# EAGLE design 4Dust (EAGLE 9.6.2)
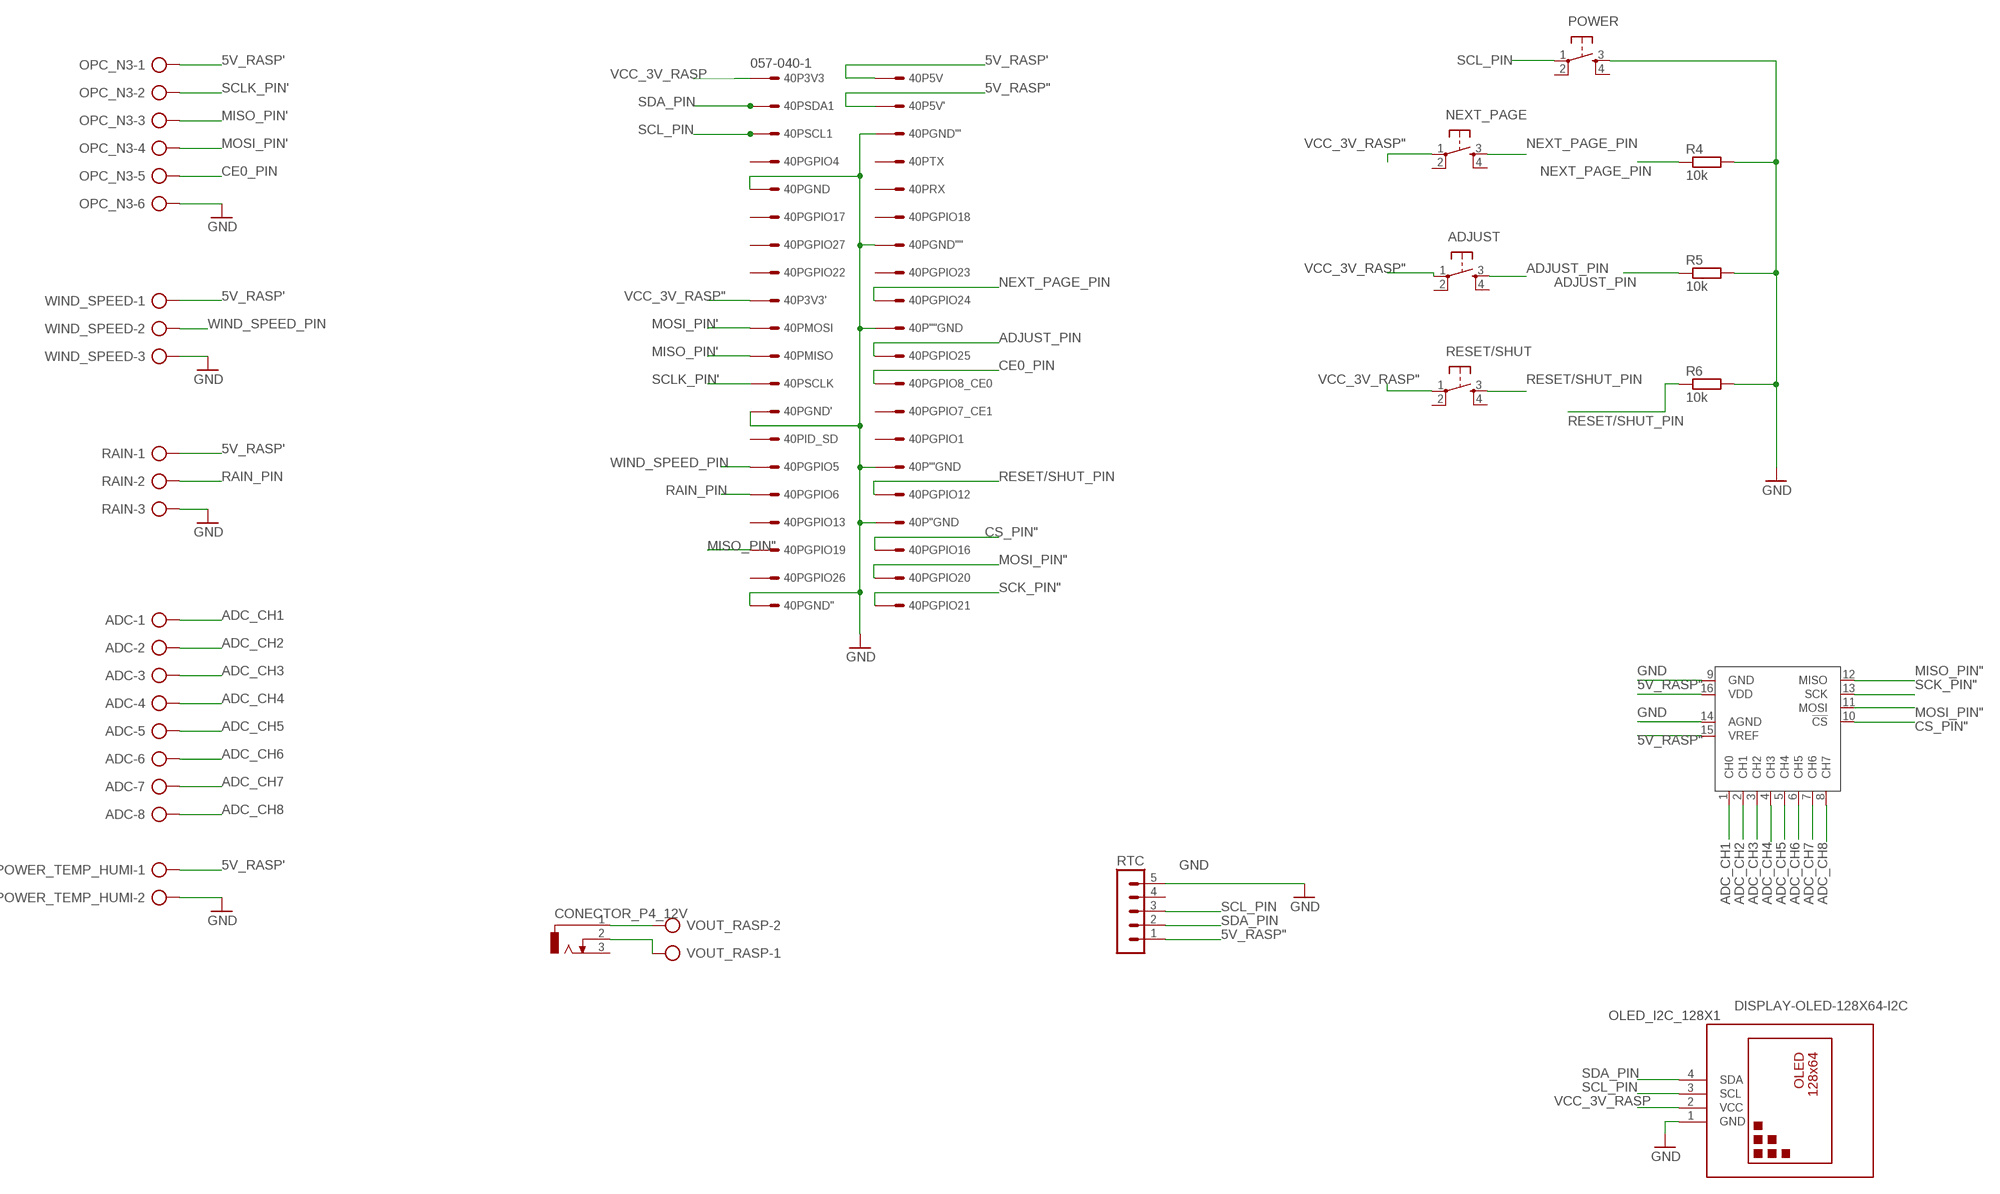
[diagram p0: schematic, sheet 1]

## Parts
40P  057-040-1  [057-040-1]
ADC  AK500/8  [AK500/8]
ADJUST  TAC_SWITCHPTH  [TACTILE-PTH]
CONECTOR_P4_12V  DCJ0303  [DCJ0303]
MCP3008  MCP3008P  [DIL16]
NEXT_PAGE  TAC_SWITCHPTH  [TACTILE-PTH]
OLED_I2C_128X1  DISPLAY-OLED-128X64-I2C  [DISPLAY-OLED-128X64-I2C]
OPC_N3  AK500/6  [AK500/6]
POWER  TAC_SWITCHPTH  [TACTILE-PTH]
POWER_TEMP_HUMI  AK500/2  [AK500/2]
R4  10k  R-EU_0204/7  [0204/7]
R5  10k  R-EU_0204/7  [0204/7]
R6  10k  R-EU_0204/7  [0204/7]
RAIN  AK500/3  [AK500/3]
RESET/SHUT  TAC_SWITCHPTH  [TACTILE-PTH]
RTC  MA05-1  [MA05-1]
VOUT_RASP  AK500/2  [AK500/2]
WIND_SPEED  AK500/3  [AK500/3]

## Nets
5V_RASP": 40P.4 MCP3008.15(VREF) MCP3008.16(VDD) RTC.1
5V_RASP': 40P.2 OPC_N3.1 POWER_TEMP_HUMI.1 RAIN.1 WIND_SPEED.1
ADC_CH1: ADC.1 MCP3008.1(CH0)
ADC_CH2: ADC.2 MCP3008.2(CH1)
ADC_CH3: ADC.3 MCP3008.3(CH2)
ADC_CH4: ADC.4 MCP3008.4(CH3)
ADC_CH5: ADC.5 MCP3008.5(CH4)
ADC_CH6: ADC.6 MCP3008.6(CH5)
ADC_CH7: ADC.7 MCP3008.7(CH6)
ADC_CH8: ADC.8 MCP3008.8(CH7)
ADJUST_PIN: 40P.22 ADJUST.3 R5.1
CE0_PIN: 40P.24 OPC_N3.5
CS_PIN": 40P.36 MCP3008.10(!CS)
GND: 40P.6 40P.9 40P.14 40P.20 40P.25 40P.30 40P.34 40P.39 MCP3008.9(GND) MCP3008.14(AGND) OLED_I2C_128X1.1(GND) OPC_N3.6 POWER.3 POWER_TEMP_HUMI.2 R4.2 R5.2 R6.2 RAIN.3 RTC.5 WIND_SPEED.3
MISO_PIN": 40P.35 MCP3008.12(MISO)
MISO_PIN': 40P.21 OPC_N3.3
MOSI_PIN": 40P.38 MCP3008.11(MOSI)
MOSI_PIN': 40P.19 OPC_N3.4
N$1: CONECTOR_P4_12V.1 VOUT_RASP.2
N$2: CONECTOR_P4_12V.2 VOUT_RASP.1
NEXT_PAGE_PIN: 40P.18 NEXT_PAGE.3 R4.1
RAIN_PIN: 40P.31 RAIN.2
RESET/SHUT_PIN: 40P.32 R6.1 RESET/SHUT.3
SCK_PIN": 40P.40 MCP3008.13(SCK)
SCL_PIN: 40P.5 OLED_I2C_128X1.3(SCL) POWER.1 RTC.3
SCLK_PIN': 40P.23 OPC_N3.2
SDA_PIN: 40P.3 OLED_I2C_128X1.4(SDA) RTC.2
VCC_3V_RASP: 40P.1 OLED_I2C_128X1.2(VCC)
VCC_3V_RASP": 40P.17 ADJUST.1 NEXT_PAGE.1 RESET/SHUT.1
WIND_SPEED_PIN: 40P.29 WIND_SPEED.2
Unconnected: 40P.7 40P.8 40P.10 40P.11 40P.12 40P.13 40P.15 40P.16 40P.26 40P.27 40P.28 40P.33 40P.37 ADJUST.2 ADJUST.4 CONECTOR_P4_12V.3 NEXT_PAGE.2 NEXT_PAGE.4 POWER.2 POWER.4 RESET/SHUT.2 RESET/SHUT.4 RTC.4

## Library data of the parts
40P = con-panduit-40pin_header:057-040-: CONNECTOR 40-pin series 057 contact pc board low profile headers; OC_FARNELL: unknown; OC_NEWARK: unknown
ADC = con-ptr500:AK500/8: CONNECTOR; OC_FARNELL: unknown; OC_NEWARK: unknown
ADJUST NEXT_PAGE POWER RESET/SHUT = SparkFun:TAC_SWITCH: Momentary Switch Button commonly used for reset or general input. Spark Fun Electronics SKU : COM-00097
CONECTOR_P4_12V = con-jack:DCJ0303: DC POWER JACK Source: DCJ0303.pdf; OC_FARNELL: unknown; OC_NEWARK: unknown
MCP3008 = MCP3008:MCP3008
OLED_I2C_128X1 = diy-modules:DISPLAY-OLED-128X64-I2C: 128x64 Dot Matrix OLED Module based on SSD1306 chip Variant with I2C interface More details available here: http://www.instructables.com/id/Monochrome-096-i2c-OLED-display-with-arduino-SSD13/ SSD1306 datasheet: https://cdn-shop.adafruit.com/datasheets/SSD1306.pdf Click here to find device on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
OPC_N3 = con-ptr500:AK500/6: CONNECTOR; OC_FARNELL: unknown; OC_NEWARK: unknown
POWER_TEMP_HUMI VOUT_RASP = con-ptr500:AK500/2: CONNECTOR; OC_FARNELL: unknown; OC_NEWARK: unknown
R4-R6 = rcl:R-EU_: RESISTOR, European symbol; SPICEPREFIX: R
RAIN WIND_SPEED = con-ptr500:AK500/3: CONNECTOR; OC_FARNELL: unknown; OC_NEWARK: unknown
RTC = con-lstb:MA05-1: PIN HEADER; OC_FARNELL: unknown; OC_NEWARK: unknown

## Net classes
0 default: clearance 0.205 mm

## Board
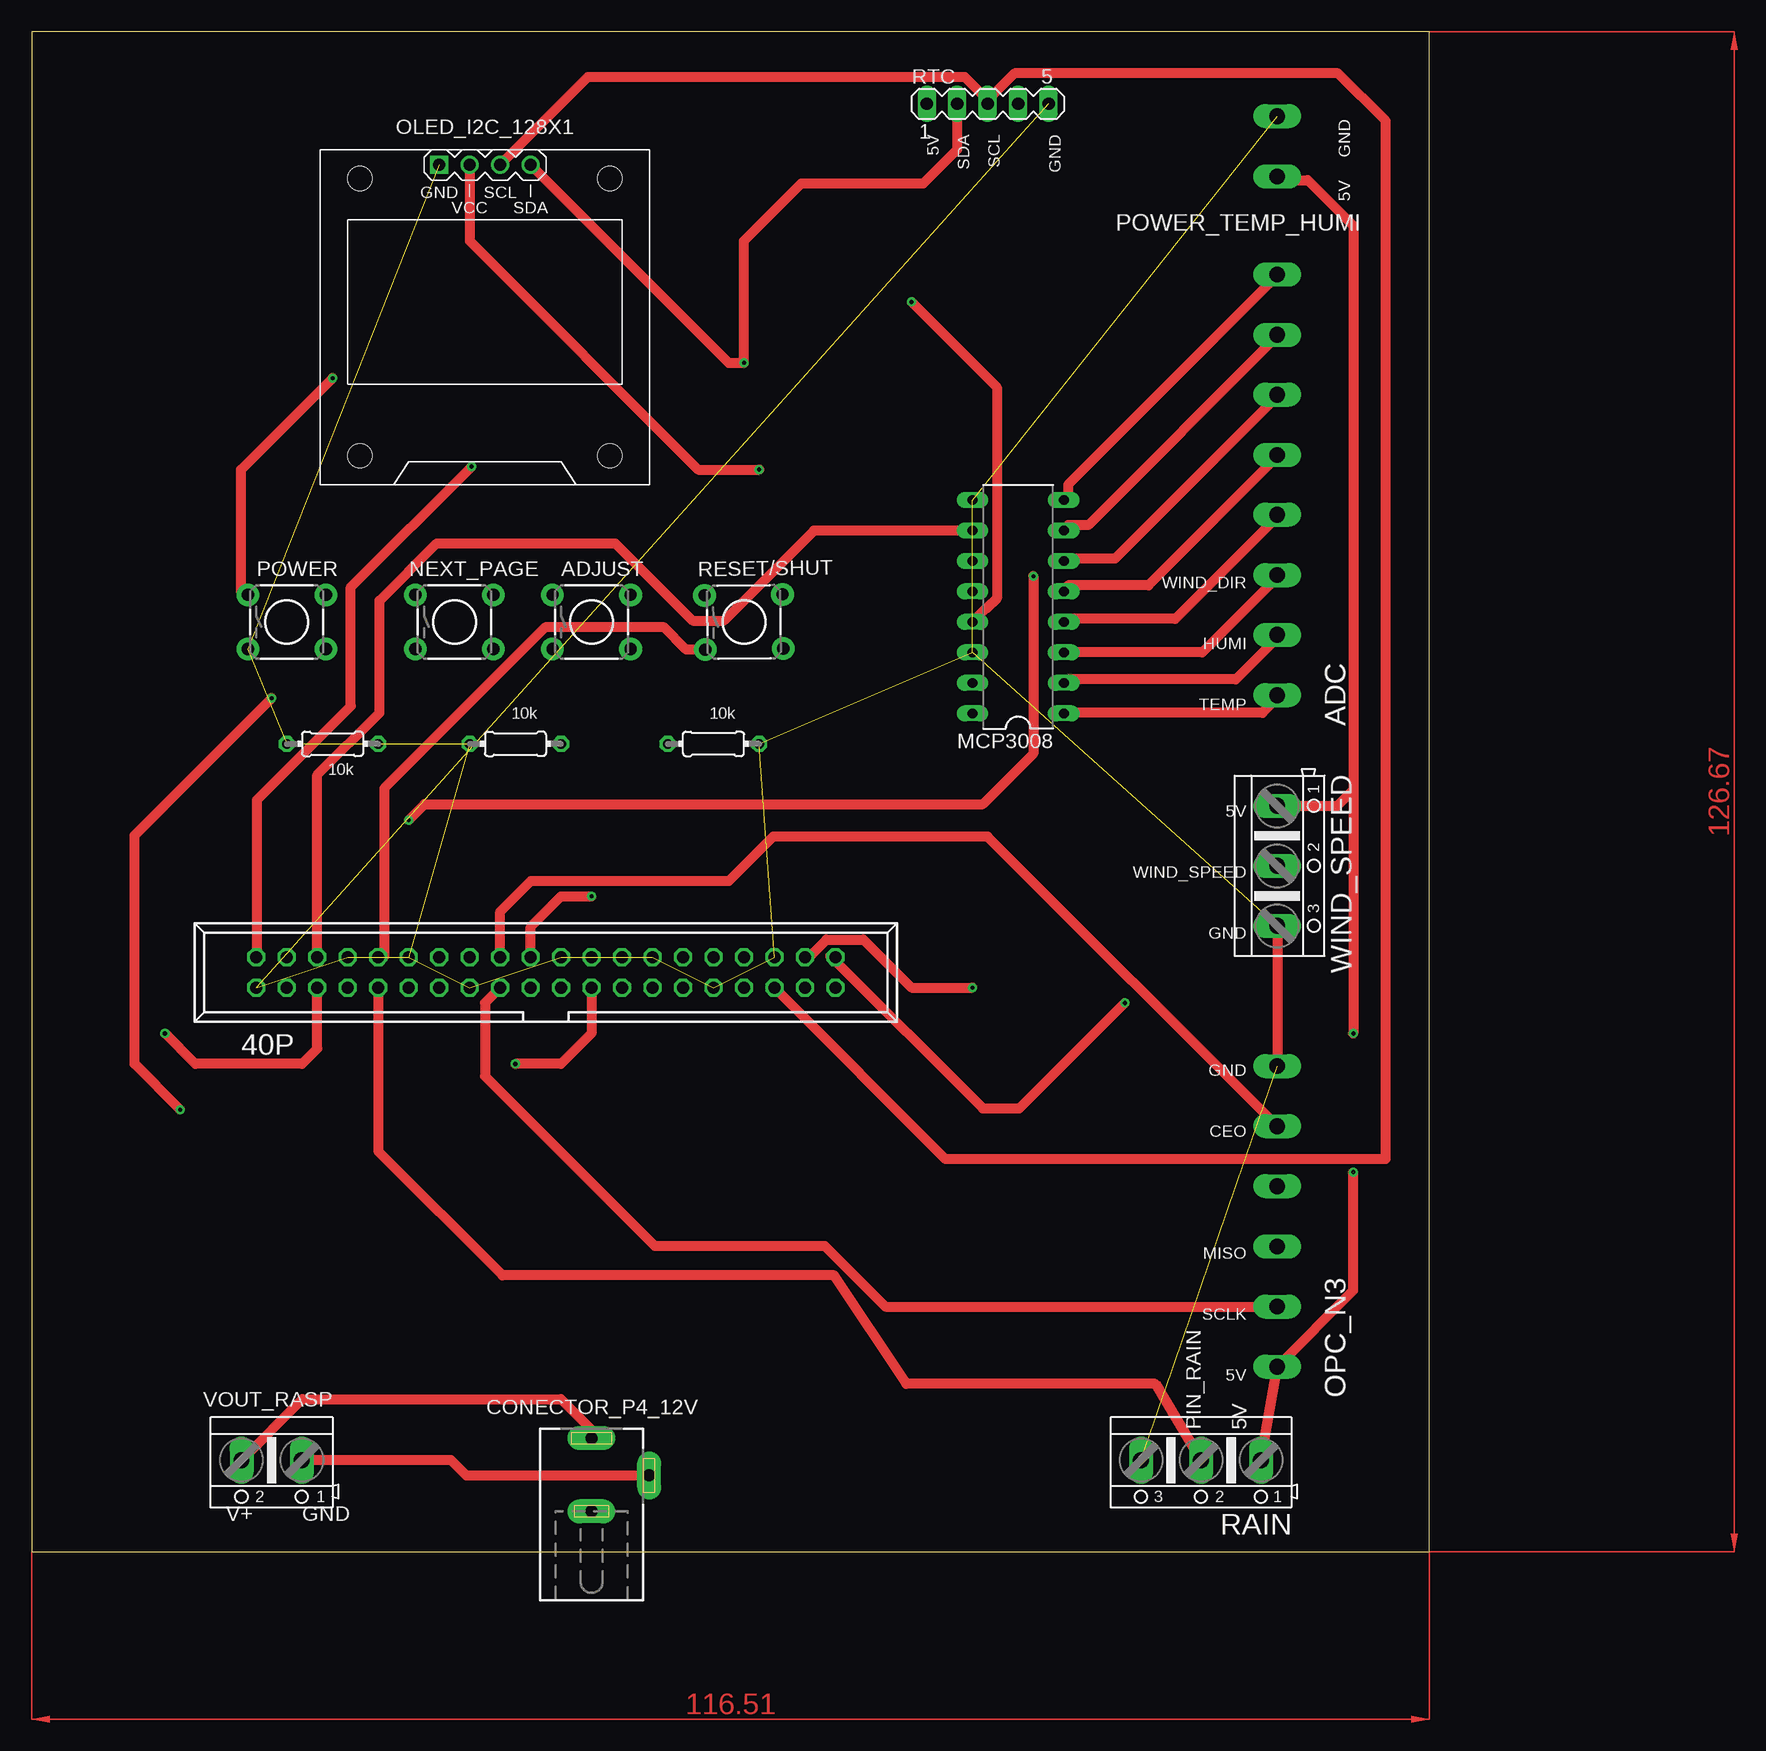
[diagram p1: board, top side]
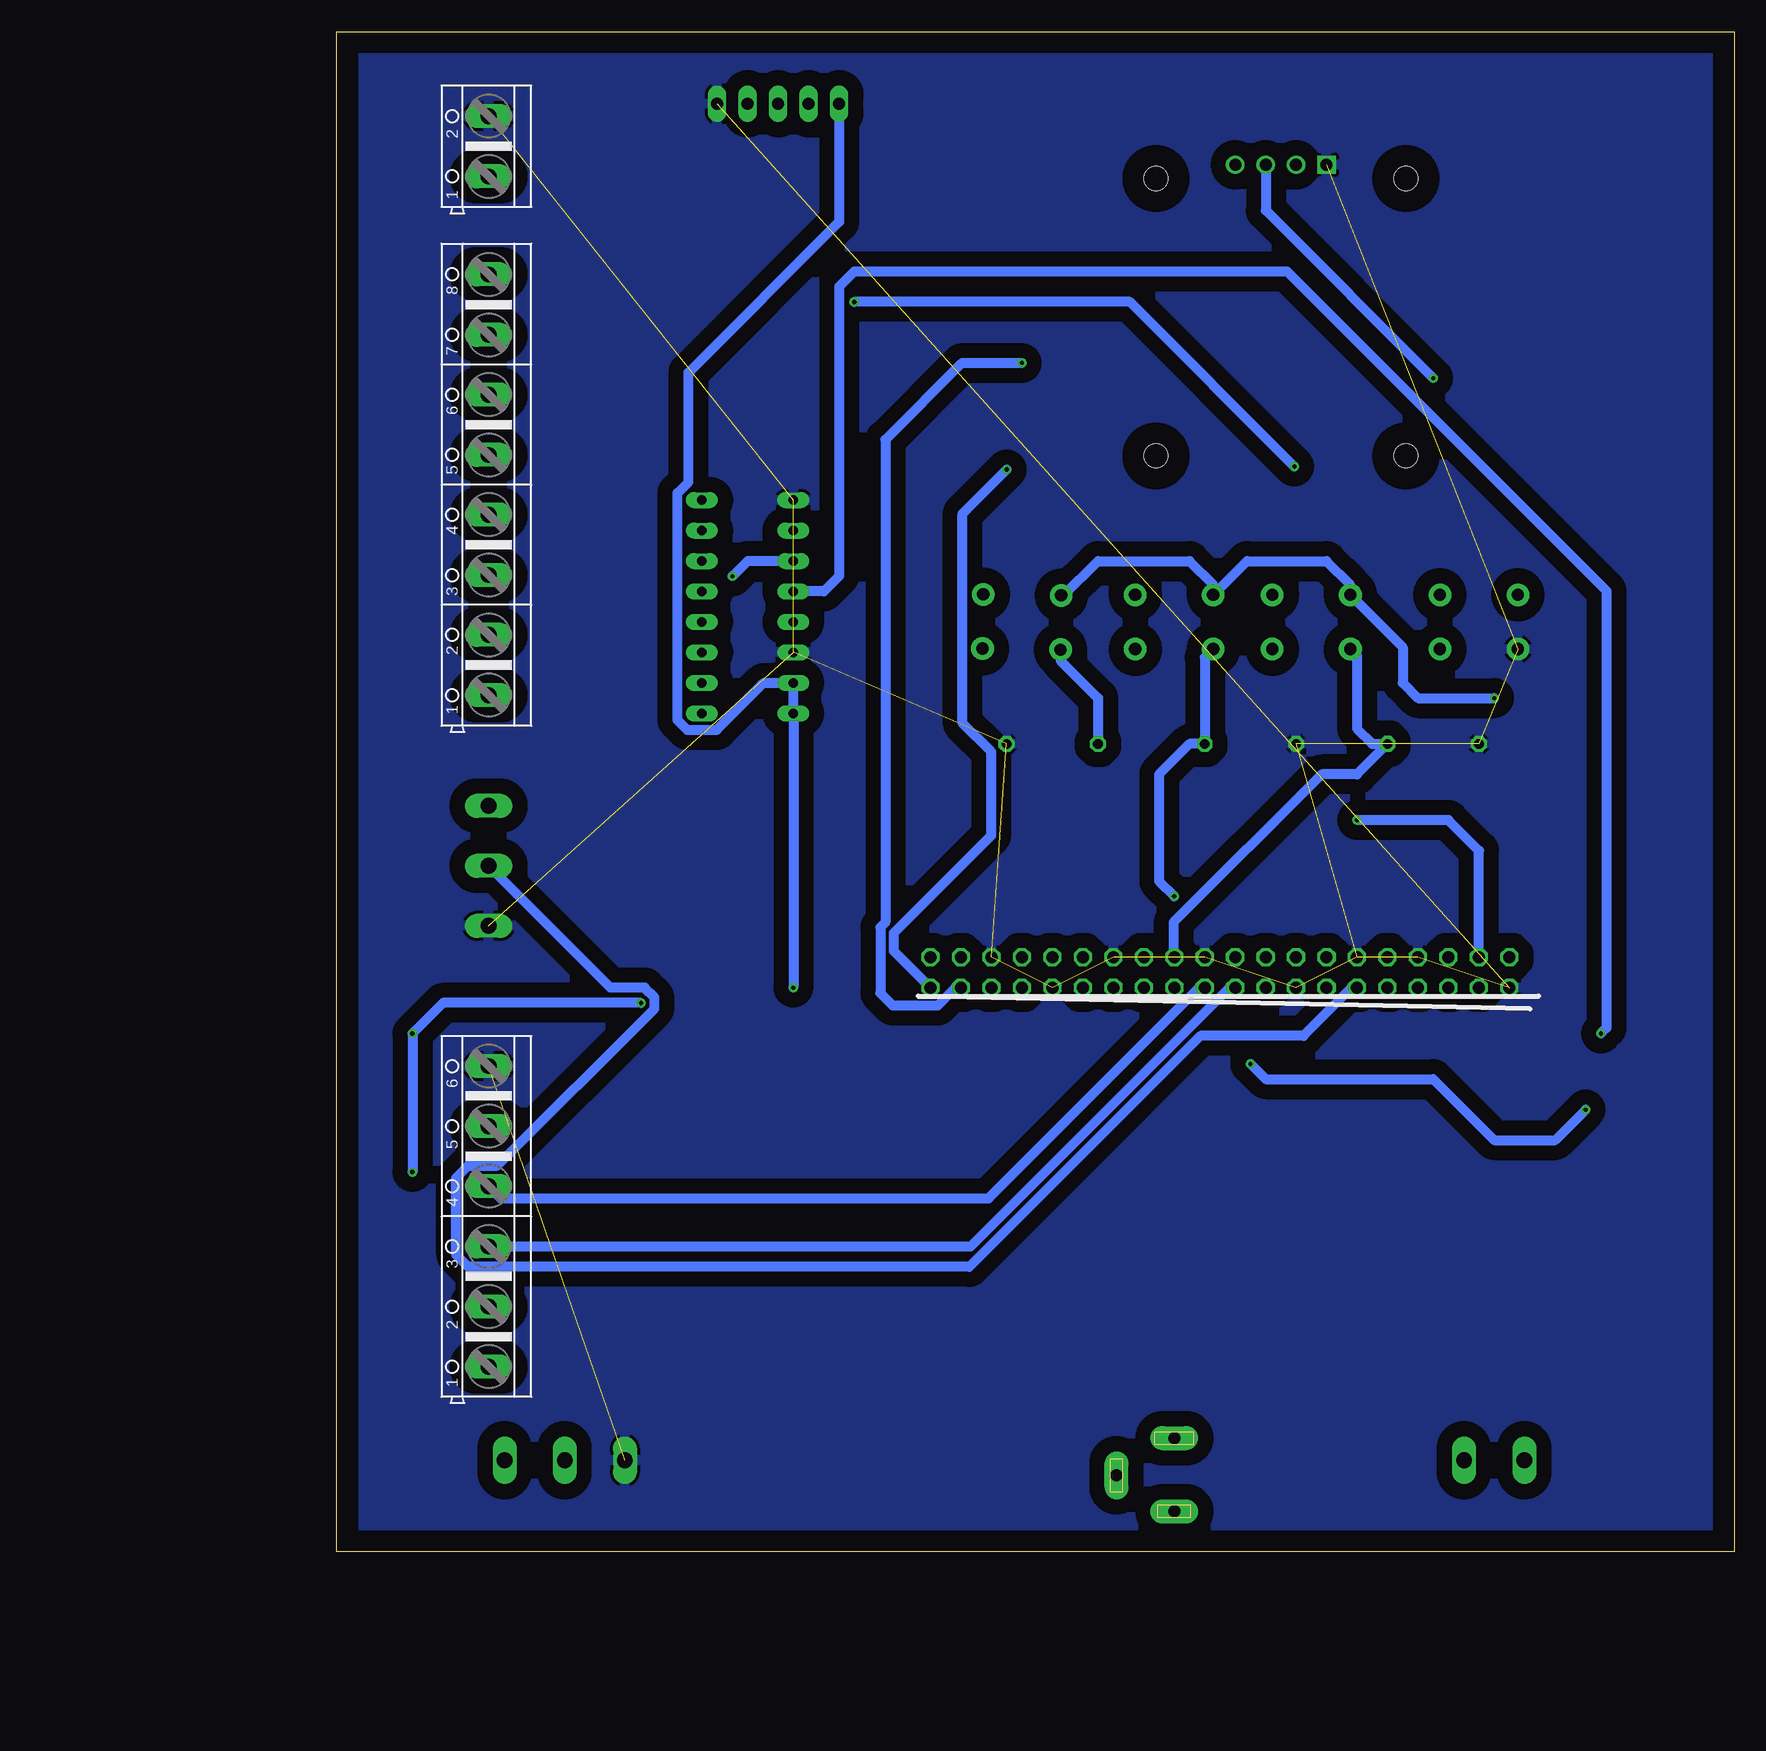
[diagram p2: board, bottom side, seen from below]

Size 116.51 x 126.67 mm. Coordinates in mm from the lower left corner, seen from the top.
Outline: 0,0 116.51,0 116.51,126.67 0,126.67 0,0
Copper layers (1*16): Top 0.035mm / dielectric 1.5mm / Bottom 0.035mm
Design rules "default *": minimum track width 32mil, minimum drill 0.35mm, track to track 12mil, track to pad 12mil, pad to pad 12mil, via to via 12mil, smd to smd 8mil, copper to edge 70mil, drill to drill 8mil, minimum pad ring 10mil, minimum via ring 8mil, stop-mask expansion 4mil, vias tented up to drill 0mil, thermal gap 10mil

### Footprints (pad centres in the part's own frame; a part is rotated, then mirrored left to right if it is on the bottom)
057-040-1 = drill 1 octagon: 1 24.13,-1.27; 2 24.13,1.27; 3 21.59,-1.27; 4 21.59,1.27; 5 19.05,-1.27; 6 19.05,1.27; 7 16.51,-1.27; 8 16.51,1.27; 9 13.97,-1.27; 10 13.97,1.27; 11 11.43,-1.27; 12 11.43,1.27; 13 8.89,-1.27; 14 8.89,1.27; 15 6.35,-1.27; 16 6.35,1.27; 17 3.81,-1.27; 18 3.81,1.27; 19 1.27,-1.27; 20 1.27,1.27; 21 -1.27,-1.27; 22 -1.27,1.27; 23 -3.81,-1.27; 24 -3.81,1.27; 25 -6.35,-1.27; 26 -6.35,1.27; 27 -8.89,-1.27; 28 -8.89,1.27; 29 -11.43,-1.27; 30 -11.43,1.27; 31 -13.97,-1.27; 32 -13.97,1.27; 33 -16.51,-1.27; 34 -16.51,1.27; 35 -19.05,-1.27; 36 -19.05,1.27; 37 -21.59,-1.27; 38 -21.59,1.27; 39 -24.13,-1.27; 40 -24.13,1.27
AK500/8 = drill 1.321 long: 1 -17.526,0; 2 -12.497,0; 3 -7.518,0; 4 -2.489,0; 5 2.489,0; 6 7.518,0; 7 12.497,0; 8 17.526,0
TACTILE-PTH = drill 1.016 pad 1.88: 1 -3.251,2.261; 2 3.251,2.261; 3 -3.251,-2.261; 4 3.251,-2.261
DCJ0303 = drill 1 pad 2 long: 1 0,3.1; 2 4.8,0; 3 0,-3
DIL16 = drill 0.813 long: 1 -8.89,-3.81; 2 -6.35,-3.81; 3 -3.81,-3.81; 4 -1.27,-3.81; 5 1.27,-3.81; 6 3.81,-3.81; 7 6.35,-3.81; 8 8.89,-3.81; 9 8.89,3.81; 10 6.35,3.81; 11 3.81,3.81; 12 1.27,3.81; 13 -1.27,3.81; 14 -3.81,3.81; 15 -6.35,3.81; 16 -8.89,3.81
DISPLAY-OLED-128X64-I2C = drill 1 square: 1 -3.81,12.7 | drill 1: 2 -1.27,12.7; 3 1.27,12.7; 4 3.81,12.7 | hole 2: -10.414,11.557; 10.414,11.557; 10.414,-11.557; -10.414,-11.557
AK500/6 = drill 1.321 long: 1 -12.522,0; 2 -7.518,0; 3 -2.515,0; 4 2.515,0; 5 7.518,0; 6 12.522,0
AK500/2 = drill 1.321 long: 1 -2.515,0; 2 2.515,0
0204/7 = drill 0.813 octagon: 1 -3.81,0; 2 3.81,0
AK500/3 = drill 1.321 long: 1 -5.004,0; 2 0,0; 3 5.004,0
MA05-1 = drill 1.016 long: 1 -5.08,0; 2 -2.54,0; 3 0,0; 4 2.54,0; 5 5.08,0

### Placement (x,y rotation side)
40P  42.87,48.26 0 top
ADC  103.83,88.9 90 bottom
ADJUST  46.68,77.47 0 top
CONECTOR_P4_12V  46.68,6.35 0 top
MCP3008  82.24,78.74 90 top
NEXT_PAGE  35.25,77.47 0 top
OLED_I2C_128X1  37.79,102.87 0 top
OPC_N3  103.83,27.94 90 bottom
POWER  21.28,77.47 0 top
POWER_TEMP_HUMI  103.83,117.11 90 bottom
R4  25.09,67.31 180 top
R5  40.33,67.31 180 top
R6  56.84,67.31 0 top
RAIN  97.48,7.62 180 top
RESET/SHUT  59.38,77.47 0.8 top
RTC  79.7,120.65 0 top
VOUT_RASP  20.01,7.62 180 top
WIND_SPEED  103.83,57.15 270 top

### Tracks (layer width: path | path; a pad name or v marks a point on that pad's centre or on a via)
5V_RASP"  (via drill 0.35)
  Top 0.813: v78.43,46.99 73.35,46.99 69.34,50.99 66.27,50.99 64.8,49.53 40P.4
  Bottom 0.813: v78.43,46.99 MCP3008.16 MCP3008.15 80.91,72.39 84.82,68.48 87.28,68.48 88.08,69.28 88.08,88.2 87.17,89.11 87.17,98.25 74.62,110.8 RTC.1
5V_RASP'  (via drill 0.35)  (1 unrouted)
  Top 0.813: 40P.2 66.59,49.63 79.29,36.93 82.34,36.93 v91.13,45.72 | POWER_TEMP_HUMI.1 104.12,114.3 106.37,114.3 110.18,110.49 110.18,63.5 | 110.18,63.5 v110.18,43.18 | RAIN.1 OPC_N3.1 110.18,21.77 110.18,31.6 | WIND_SPEED.1 108.83,62.15 110.18,63.5
  Bottom 0.813: v91.13,45.72 107.64,45.72 v110.18,43.18 v110.18,31.63
ADC_CH1
  Top 0.813: MCP3008.1 86.41,69.9 102.61,69.9 103.73,71.02 ADC.1
ADC_CH2
  Top 0.813: MCP3008.2 86.41,72.69 100.38,72.69 103.73,76.05 ADC.2
ADC_CH3
  Top 0.813: MCP3008.3 97.58,74.93 103.73,81.08 ADC.3
ADC_CH4
  Top 0.813: MCP3008.4 86.41,77.72 95.35,77.72 103.73,86.11 ADC.4
ADC_CH5
  Top 0.813: MCP3008.5 86.41,80.52 93.11,80.52 103.73,91.14 ADC.5
ADC_CH6
  Top 0.813: MCP3008.6 86.41,82.75 90.32,82.75 103.73,96.16 ADC.6
ADC_CH7
  Top 0.813: MCP3008.7 86.41,85.55 88.08,85.55 103.73,101.19 ADC.7
ADC_CH8
  Top 0.813: MCP3008.8 86.41,87.78 86.41,88.9 103.73,106.22 ADC.8
ADJUST_PIN  (via drill 0.35)
  Top 0.813: 40P.22 41.6,52.07 44.14,54.61 v46.68,54.61
  Bottom 0.813: ADJUST.3 44.14,74.5 R5.1 45.41,67.31 47.95,64.77 47.95,55.88 v46.68,54.61
CE0_PIN
  Top 0.813: OPC_N3.5 79.7,59.59 61.82,59.59 58.11,55.88 41.6,55.88 39.06,53.34 40P.24
CS_PIN"
  Top 0.813: MCP3008.10 65.22,85.09 57.7,77.57 55.11,77.57 48.66,84.02 33.78,84.02 29,79.25 29,69.9 23.82,64.72 40P.36
GND  (18 unrouted)
  Top 0.813: WIND_SPEED.3 OPC_N3.6
  pour Bottom (isolate 1.27): 1,125.73 115.26,125.73 115.26,1.27 1,1.27
MISO_PIN"  (via drill 0.35)
  Top 0.813: 40P.35 23.82,41.91 22.55,40.64 13.66,40.64 v11.12,43.18
  Bottom 0.813: MCP3008.12 75.89,80.01 74.62,81.28 74.62,105.41 73.35,106.68 37.28,106.68 10.66,80.06 10.66,43.64 v11.12,43.18
MISO_PIN'
  Bottom 0.813: OPC_N3.3 63.63,25.43 42.07,46.99 40P.21
MOSI_PIN"  (via drill 0.35)
  Top 0.813: v31.44,60.96 32.76,62.28 79.29,62.28 83.51,66.5 v83.51,81.28
  Bottom 0.813: 40P.38 21.28,58.42 23.82,60.96 v31.44,60.96 | MCP3008.11 82.24,82.55 v83.51,81.28
MOSI_PIN'
  Bottom 0.813: 40P.19 44.09,46.95 44.65,46.95 62.15,29.44 102.82,29.44 OPC_N3.4
N$1
  Top 0.813: VOUT_RASP.2 22.58,12.7 44.14,12.7 46.68,10.16 CONECTOR_P4_12V.1
N$2
  Top 0.813: CONECTOR_P4_12V.2 36.24,6.35 34.97,7.62 VOUT_RASP.1
NEXT_PAGE_PIN
  Bottom 0.813: 40P.18 46.73,49.63 46.73,52.43 34.39,64.77 31.44,64.77 R4.1 30.17,67.31 31.44,68.58 31.44,74.65 NEXT_PAGE.3
RAIN_PIN
  Top 0.813: 40P.31 28.9,33.38 39.26,23.01 66.9,23.01 72.93,13.97 93.67,13.97 RAIN.2
RESET/SHUT_PIN
  Top 0.813: 40P.32 29.41,49.63 29.41,63.6 42.82,77.01 52.72,77.01 54.57,75.16 RESET/SHUT.3
  Bottom 0.813: RESET/SHUT.3 56.16,74.25 53.03,71.12 R6.1
SCK_PIN"  (via drill 0.35)
  Top 0.813: v36.67,90.42 26.61,80.37 26.61,70.46 18.79,62.64 18.79,49.63 40P.40 | MCP3008.13 79.6,78.64 79.66,78.64 80.46,79.44 80.46,97.03 v73.35,104.14
  Bottom 0.813: v73.35,104.14 50.39,104.14 v36.67,90.42
SCL_PIN  (via drill 0.35)
  Top 0.813: 40P.5 76.19,32.72 112.87,32.72 112.87,119.23 108.91,123.19 81.94,123.19 79.55,120.8 RTC.3 79.85,120.8 77.77,122.89 46.38,122.89 OLED_I2C_128X1.3 | POWER.1 17.75,79.73 17.47,80.01 17.47,90.17 v25.09,97.79
  Bottom 0.813: OLED_I2C_128X1.3 39.06,111.76 v25.09,97.79
SCLK_PIN'
  Top 0.813: 40P.23 37.79,45.72 37.79,39.62 51.95,25.47 66.12,25.47 71.17,20.42 OPC_N3.2
SDA_PIN  (via drill 0.35)
  Top 0.813: OLED_I2C_128X1.4 58.11,99.06 v59.38,99.06 59.38,109.22 64.16,114 74.31,114 77.16,116.84 RTC.2
  Bottom 0.813: v59.38,99.06 64.36,99.06 70.76,92.66 70.76,52.43 71.17,52.02 71.17,46.54 70.15,45.52 66.39,45.52 64.93,46.99 40P.3
VCC_3V_RASP  (via drill 0.35)
  Top 0.813: OLED_I2C_128X1.2 36.52,109.22 55.57,90.17 v60.65,90.17
  Bottom 0.813: 40P.1 70.05,50.04 70.05,51.56 61.92,59.69 61.92,66.64 64.32,69.04 64.32,86.5 v60.65,90.17
VCC_3V_RASP"  (via drill 0.35)
  Top 0.813: 40P.17 46.68,43.18 44.14,40.64 v40.33,40.64 | v12.39,36.83 8.58,40.64 8.58,59.69 v20.01,71.12
  Bottom 0.813: RESET/SHUT.1 55.89,79.69 53.03,82.55 45.41,82.55 43.43,80.57 ADJUST.1 40.61,82.55 33.98,82.55 32,80.57 NEXT_PAGE.1 27.63,75.36 27.63,72.39 26.36,71.12 v20.01,71.12 | v40.33,40.64 39.06,39.37 25.09,39.37 20.01,34.29 14.93,34.29 v12.39,36.83
WIND_SPEED_PIN
  Bottom 0.813: WIND_SPEED.2 93.67,46.99 90.82,46.99 90.01,46.18 90.01,45.26 103.11,32.16 105.53,32.16 106.52,31.16 106.52,24.72 105.53,23.72 63.75,23.72 44.49,42.98 35.91,42.98 31.91,46.99 40P.29
(copper drawn outside any net)
  shapes: Top area x2

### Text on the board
tNames: GND | 5V | SDA | SCL | GND | 5V | POWER | WIND_DIR | HUMI | TEMP | 5V | WIND_SPEED | GND | GND | CEO | MISO | SCLK | 5V | PIN_RAIN | 5V | V+ | GND
tValues: MOSI

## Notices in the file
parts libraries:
diy-modules: Released under the Creative Commons Attribution 4.0 International License: http://creativecommons.org/licenses/by/4.0
SparkFun: Licensing: CC v3.0 Share-Alike You are welcome to use this library for commercial purposes.
